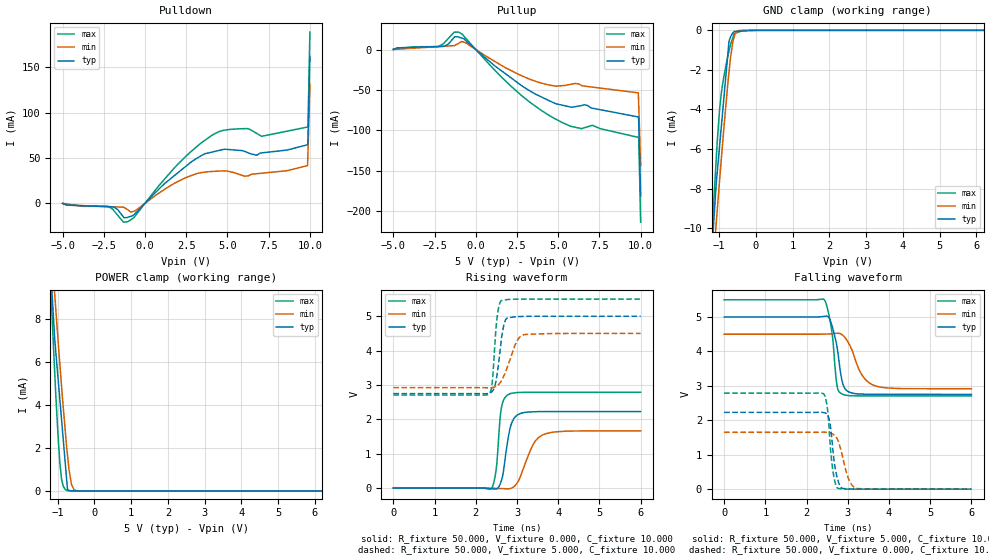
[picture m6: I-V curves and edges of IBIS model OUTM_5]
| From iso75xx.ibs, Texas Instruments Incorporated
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|   OUTM_5 MODEL
[Model]   OUTM_5
Model_type   3-state
Polarity   Non-Inverting
Vmeas = 2.5
Vref = 2.5
Cref = 15pF
Rref = 50
|   typ   min   max
| High state   (typ PVT)   (Fast PVT)  (Slow PVT)
C_comp   1.5194p   1.2464p   1.8503p
|C_comp (Low state)   1.4779p   1.2343p   1.7765p
[Voltage Range]   5   4.5   5.5
[Temperature Range]   27   125   -40
[Pullup Reference]   5   4.5   5.5
[Pulldown Reference]   -0   -0   -0
[Power Clamp Reference]   5   4.5   5.5
[GND Clamp Reference]   -0   -0   -0
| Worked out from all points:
|   slope of the pulldown table from 0 to 0.75 V, typ, clamps not added: 53.7 ohm
|   slope of the pullup table from 0 to 0.75 V, typ, clamps not added: 56.6 ohm
|   GND clamp passes 1 mA (typ) near -0.75 V on its own axis
|   POWER clamp passes 1 mA (typ) near -0.78 V on its own axis
|   falling waveform, R_fixture 50.000, V_fixture 5.000, C_fixture 10.000: 20-80 % time 190ps typ, 347ps min, 149ps max; typ from 5 V to 2.75 V
|   rising waveform, R_fixture 50.000, V_fixture 0.000, C_fixture 10.000: 20-80 % time 175ps typ, 344ps min, 112ps max; typ from 0 V to 2.23 V
|   rising waveform, R_fixture 50.000, V_fixture 5.000, C_fixture 10.000: 20-80 % time 147ps typ, 292ps min, 101ps max; typ from 2.75 V to 5 V
|   falling waveform, R_fixture 50.000, V_fixture 0.000, C_fixture 10.000: 20-80 % time 136ps typ, 217ps min, 121ps max; typ from 2.23 V to 0 V
[Pulldown]
|   Voltage   I(typ)   I(min)   I(max)
-5V       -142.9uA   -109.4uA   -135.2uA
-2.283V   -3.758mA   -3.68mA    -3.416mA
-1.053V   -15.54mA   -7.054mA   -20.38mA
-623.8mV  -11.88mA   -8.605mA   -14.57mA
2.816V    45.87mA    30.63mA    57.52mA
4.174V    56.97mA    35.23mA    76.28mA
6.026V    57.41mA    30mA       82.38mA
7.07V     55.59mA    33.16mA    73.9mA
8.601V    58.73mA    35.91mA    79.55mA
9.86V     64.62mA    41.62mA    84.21mA
9.884V    71.61mA    56.7mA     84.29mA
10V       162.2mA    131.2mA    189mA
[GND Clamp]
|   Voltage   I(typ)   I(min)   I(max)
-5V       -95.55mA   -83.03mA   -109.1mA
-1.902V   -31.92mA   -29.32mA   -36.05mA
-1.157V   -10.01mA   -11.6mA    -9.009mA
-1.081V   -7.777mA   -9.793mA   -6.565mA
-984.6mV  -5.787mA   -7.529mA   -3.942mA
-938.9mV  -4.841mA   -6.48mA    -3.154mA
-731.6mV  -551.3uA   -2.119mA   -1.051mA
-623.8mV  -130.8uA   -538.2uA   -355.5uA
-582.4mV  -52.36uA   -283.9uA   -168uA
-491.8mV  -44.9uA    -25uA      -104.8uA
-342.3mV  -32.57uA   -484.6nA   -520.1nA
10V       0A         0A         0A
[Pullup]
|   Voltage   I(typ)   I(min)   I(max)
-5V       146.7uA    117.7uA    151.3uA
-2.329V   3.698mA    3.49mA     3.506mA
-1.053V   15.45mA    7.463mA    21.54mA
-623.8mV  11.35mA    8.47mA     14.26mA
2.103V    -34.48mA   -25.64mA   -44.72mA
4.44V     -63.09mA   -43.77mA   -81.26mA
5.749V    -71.08mA   -43.04mA   -94.81mA
7.07V     -72.48mA   -46.45mA   -93.64mA
9.86V     -83.38mA   -53.56mA   -108.6mA
9.875V    -83.43mA   -62.92mA   -108.6mA
9.884V    -90.33mA   -68.59mA   -108.7mA
10V       -180.8mA   -142.8mA   -213.4mA
[POWER Clamp]
|   Voltage   I(typ)   I(min)   I(max)
-5V       95.31mA    82.73mA    108.9mA
-1.902V   31.32mA    28.72mA    35.43mA
-1.081V   7.105mA    9.192mA    5.566mA
-984.6mV  5.167mA    6.936mA    2.444mA
-938.9mV  4.245mA    5.898mA    1.296mA
-893.2mV  3.324mA    4.877mA    551.9uA
-847.5mV  2.402mA    3.908mA    220.8uA
-756mV    559uA      2.06mA     29.16uA
-731.6mV  67.22uA    1.666mA    19.98uA
-623.8mV  4.585uA    311.6uA    1.77uA
-491.8mV  3.69uA     9.862uA    117.9nA
10V       0A         0A         0A
[Ramp]
R_load = 50
|   typ   min   max
dV/dt_r   1.35465/1.75359e-10   0.998976/3.44388e-10   1.69935/1.12135e-10
dV/dt_f   1.36762/1.89405e-10   0.950504/3.47364e-10   1.70152/1.49212e-10
[Falling Waveform]
R_fixture = 50.000
V_fixture = 5.000
V_fixture_min = 4.500
V_fixture_max = 5.500
C_fixture = 10.000
|  time   V(typ)   V(min)   V(max)
0s        5V         4.5V       5.5V
2.414ns   5.016V     4.503V     5.516V
2.528ns   5.001V     4.507V     5.144V
2.64ns    4.653V     4.517V     4.318V
2.738ns   4.136V     4.527V     3.014V
2.875ns   3.086V     4.473V     2.754V
3.005ns   2.837V     4.274V     2.72V
3.348ns   2.761V     3.31V      2.708V
3.588ns   2.754V     3.039V     2.708V
6ns       2.753V     2.916V     2.708V
[Rising Waveform]
R_fixture = 50.000
V_fixture = 0.000
V_fixture_min = 0.000
V_fixture_max = 0.000
C_fixture = 10.000
|  time   V(typ)   V(min)   V(max)
0s        -364.4uV   3.686nV    43.14uV
2.368ns   -15.02mV   -1.723mV   -26.65mV
2.489ns   -25.15mV   -6.203mV   498.9mV
2.592ns   118.5mV    -11.46mV   2.071V
2.633ns   269mV      -13.56mV   2.407V
2.828ns   1.722V     -13.45mV   2.744V
3.042ns   2.15V      228.5mV    2.782V
3.391ns   2.22V      1.269V     2.787V
3.658ns   2.227V     1.565V     2.787V
6ns       2.227V     1.665V     2.788V
[Rising Waveform]
R_fixture = 50.000
V_fixture = 5.000
V_fixture_min = 4.500
V_fixture_max = 5.500
C_fixture = 10.000
|  time   V(typ)   V(min)   V(max)
0s        2.749V     2.924V     2.708V
2.314ns   2.755V     2.918V     2.738V
2.395ns   2.812V     2.924V     3.037V
2.484ns   3.078V     2.958V     4.556V
2.553ns   3.637V     3.014V     5.244V
2.628ns   4.39V      3.138V     5.457V
2.738ns   4.929V     3.438V     5.481V
2.985ns   4.985V     4.245V     5.498V
3.141ns   4.994V     4.456V     5.499V
6ns       5V         4.5V       5.5V
[Falling Waveform]
R_fixture = 50.000
V_fixture = 0.000
V_fixture_min = 0.000
V_fixture_max = 0.000
C_fixture = 10.000
|  time   V(typ)   V(min)   V(max)
0s        2.23V      1.652V     2.788V
2.414ns   2.224V     1.655V     2.768V
2.511ns   2.155V     1.646V     2.295V
2.567ns   1.926V     1.632V     1.414V
2.652ns   986.6mV    1.587V     440.2mV
2.757ns   270.8mV    1.425V     26.04mV
2.86ns    29.16mV    1.012V     8mV
3.017ns   6.97mV     301.2mV    2.097mV
3.176ns   1.758mV    40.98mV    459.2uV
6ns       3.446nV    -14.87nV   4.787nV
